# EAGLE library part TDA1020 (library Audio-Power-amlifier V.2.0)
The TDA1020 is a monolithic integrated 12 W audio amplifier in a 9-lead single in-line (SIL) plastic package. The device is primarily developed as a car radio amplifier. At a supply voltage of VP = 14,4 V, an output power of 7 W can be delivered into a 4 W load and 12 W into 2 W.
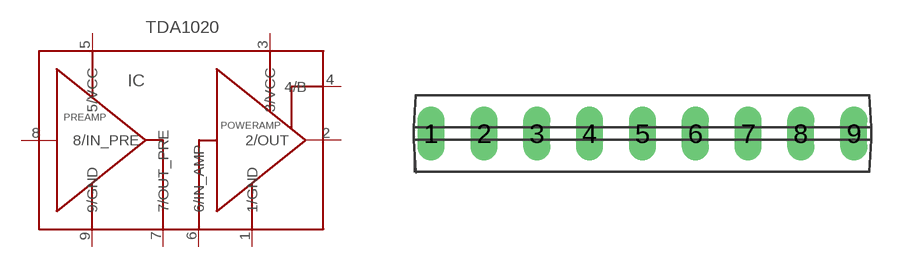
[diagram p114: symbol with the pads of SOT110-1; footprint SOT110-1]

Designator prefix IC

## TDA1020  [SOT110-1]
1  1/GND  pwr
2  2/OUT  out
3  3/VCC  pwr
4  4/B
5  5/VCC  pwr
6  6/IN_AMP  in
7  7/OUT_PRE  out
8  8/IN_PRE  in
9  9/GND  pwr

## Footprint SOT110-1 (pad centres in mm)
SIL9MPF: plastic single in-line medium power package with fin; 9 leads
drill 0.8 long: 1 -10.16,0; 2 -7.62,0; 3 -5.08,0; 4 -2.54,0; 5 0,0; 6 2.54,0; 7 5.08,0; 8 7.62,0; 9 10.16,0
